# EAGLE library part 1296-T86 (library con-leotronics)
1.27mm SINGLE ROW FEMALE SOCKET Source: http://www.leotronics.co.uk/Conexcon/Data%20Sheets/sec.%20A/1296ing.pdf
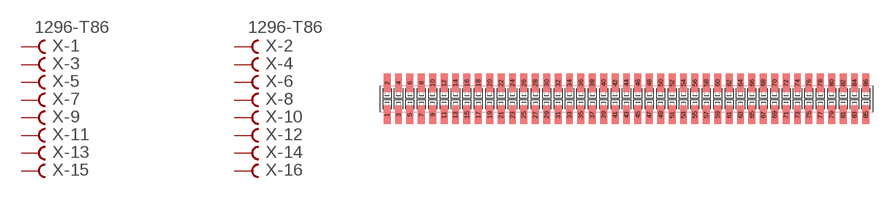
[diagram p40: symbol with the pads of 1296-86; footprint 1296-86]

Designator prefix X; gates -1=FVAL -2=FVAL -3=F -4=F -5=F -6=F -7=F -8=F -9=F -10=F -11=F -12=F -13=F -14=F -15=F -16=F -17=F -18=F -19=F -20=F -21=F -22=F -23=F -24=F -25=F -26=F -27=F -28=F -29=F -30=F -31=F -32=F -33=F -34=F -35=F -36=F -37=F -38=F -39=F -40=F -41=F -42=F -43=F -44=F -45=F -46=F -47=F -48=F -49=F -50=F -51=F -52=F -53=F -54=F -55=F -56=F -57=F -58=F -59=F -60=F -61=F -62=F -63=F -64=F -65=F -66=F -67=F -68=F -69=F -70=F -71=F -72=F -73=F -74=F -75=F -76=F -77=F -78=F -79=F -80=F -81=F -82=F -83=F -84=F -85=F -86=F

## 1296-T86 (OC_FARNELL: unknown; OC_NEWARK: unknown)  [1296-86]
1  -1:B  pas
2  -2:B  pas
3  -3:B  pas
4  -4:B  pas
5  -5:B  pas
6  -6:B  pas
7  -7:B  pas
8  -8:B  pas
9  -9:B  pas
10  -10:B  pas
11  -11:B  pas
12  -12:B  pas
13  -13:B  pas
14  -14:B  pas
15  -15:B  pas
16  -16:B  pas
17  -17:B  pas
18  -18:B  pas
19  -19:B  pas
20  -20:B  pas
21  -21:B  pas
22  -22:B  pas
23  -23:B  pas
24  -24:B  pas
25  -25:B  pas
26  -26:B  pas
27  -27:B  pas
28  -28:B  pas
29  -29:B  pas
30  -30:B  pas
31  -31:B  pas
32  -32:B  pas
33  -33:B  pas
34  -34:B  pas
35  -35:B  pas
36  -36:B  pas
37  -37:B  pas
38  -38:B  pas
39  -39:B  pas
40  -40:B  pas
41  -41:B  pas
42  -42:B  pas
43  -43:B  pas
44  -44:B  pas
45  -45:B  pas
46  -46:B  pas
47  -47:B  pas
48  -48:B  pas
49  -49:B  pas
50  -50:B  pas
51  -51:B  pas
52  -52:B  pas
53  -53:B  pas
54  -54:B  pas
55  -55:B  pas
56  -56:B  pas
57  -57:B  pas
58  -58:B  pas
59  -59:B  pas
60  -60:B  pas
61  -61:B  pas
62  -62:B  pas
63  -63:B  pas
64  -64:B  pas
65  -65:B  pas
66  -66:B  pas
67  -67:B  pas
68  -68:B  pas
69  -69:B  pas
70  -70:B  pas
71  -71:B  pas
72  -72:B  pas
73  -73:B  pas
74  -74:B  pas
75  -75:B  pas
76  -76:B  pas
77  -77:B  pas
78  -78:B  pas
79  -79:B  pas
80  -80:B  pas
81  -81:B  pas
82  -82:B  pas
83  -83:B  pas
84  -84:B  pas
85  -85:B  pas
86  -86:B  pas

## Footprint 1296-86 (pad centres in mm)
1.27mm SINGLE ROW FEMALE SOCKET Source: http://www.leotronics.co.uk/Conexcon/Data%20Sheets/sec.%20A/1296ing.pdf
smd 0.76 x 2.05: 1 -26.67,-1.78; 2 -26.67,1.78; 3 -25.4,-1.78; 4 -25.4,1.78; 5 -24.13,-1.78; 6 -24.13,1.78; 7 -22.86,-1.78; 8 -22.86,1.78; 9 -21.59,-1.78; 10 -21.59,1.78; 11 -20.32,-1.78; 12 -20.32,1.78; 13 -19.05,-1.78; 14 -19.05,1.78; 15 -17.78,-1.78; 16 -17.78,1.78; 17 -16.51,-1.78; 18 -16.51,1.78; 19 -15.24,-1.78; 20 -15.24,1.78; 21 -13.97,-1.78; 22 -13.97,1.78; 23 -12.7,-1.78; 24 -12.7,1.78; 25 -11.43,-1.78; 26 -11.43,1.78; 27 -10.16,-1.78; 28 -10.16,1.78; 29 -8.89,-1.78; 30 -8.89,1.78; 31 -7.62,-1.78; 32 -7.62,1.78; 33 -6.35,-1.78; 34 -6.35,1.78; 35 -5.08,-1.78; 36 -5.08,1.78; 37 -3.81,-1.78; 38 -3.81,1.78; 39 -2.54,-1.78; 40 -2.54,1.78; 41 -1.27,-1.78; 42 -1.27,1.78; 43 0,-1.78; 44 0,1.78; 45 1.27,-1.78; 46 1.27,1.78; 47 2.54,-1.78; 48 2.54,1.78; 49 3.81,-1.78; 50 3.81,1.78; 51 5.08,-1.78; 52 5.08,1.78; 53 6.35,-1.78; 54 6.35,1.78; 55 7.62,-1.78; 56 7.62,1.78; 57 8.89,-1.78; 58 8.89,1.78; 59 10.16,-1.78; 60 10.16,1.78; 61 11.43,-1.78; 62 11.43,1.78; 63 12.7,-1.78; 64 12.7,1.78; 65 13.97,-1.78; 66 13.97,1.78; 67 15.24,-1.78; 68 15.24,1.78; 69 16.51,-1.78; 70 16.51,1.78; 71 17.78,-1.78; 72 17.78,1.78; 73 19.05,-1.78; 74 19.05,1.78; 75 20.32,-1.78; 76 20.32,1.78; 77 21.59,-1.78; 78 21.59,1.78; 79 22.86,-1.78; 80 22.86,1.78; 81 24.13,-1.78; 82 24.13,1.78; 83 25.4,-1.78; 84 25.4,1.78; 85 26.67,-1.78; 86 26.67,1.78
